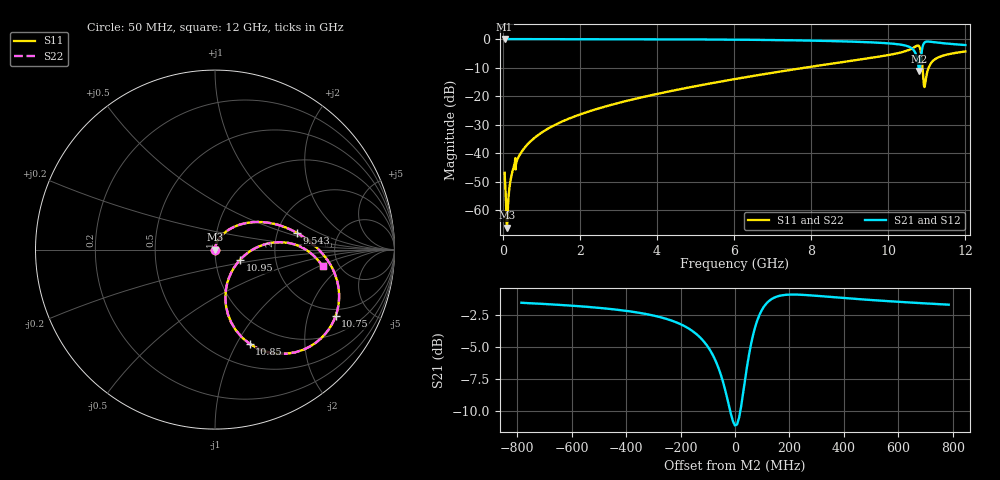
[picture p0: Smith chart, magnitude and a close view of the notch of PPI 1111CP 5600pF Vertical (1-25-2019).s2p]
# GHz S MA R 50
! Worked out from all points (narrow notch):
!   1601 points, 50 MHz to 12 GHz, reference 50 ohm
!   highest |S21| = 0.00 dB at 50 MHz (marker M1); lowest = -11.2 dB at 10.8 GHz (marker M2)
!   notch at M2: 11.0 dB deep, 131 MHz wide at half that depth
!   lowest |S11| = -66.1 dB at 109.8 MHz (marker M3), VSWR 1.00, Z = 50 - j0.0075 ohm
!   |S11| at or under -10 dB: start of sweep to 7.847 GHz; 10.89 GHz to 11.05 GHz (159.7 MHz wide, 1.46 % of centre)
!   |S22| runs from -66.1 to -2.2 dB; largest |S21 - S12| = 0
!   S11 on the Smith chart (normalised r, x): 50 MHz: 1.00, -0.01; 9.543 GHz: 2.59, +0.61; 10.75 GHz: 1.67, -3.02; 10.85 GHz: 0.74, -1.13; 10.95 GHz: 1.31, -0.16; 12 GHz: 3.74, -1.11
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0.05  0.00455 -85.4  0.9996 -0.0  0.9996 -0.0  0.00455 -85.4
0.10975  0.0004975 -8.7  0.9995 -0.6  0.9995 -0.6  0.0004975 -8.7
0.1545625  0.001804 70.8  0.9994 -1.0  0.9994 -1.0  0.001804 70.8
0.2068437  0.003451 78.0  0.9993 -1.4  0.9993 -1.4  0.003451 78.0
0.2665938  0.005178 80.2  0.9993 -1.8  0.9993 -1.8  0.005178 80.2
0.6026875  0.01331 81.5  0.9989 -4.2  0.9989 -4.2  0.01331 81.5
1.162844  0.02669 79.0  0.9982 -8.1  0.9982 -8.1  0.02669 79.0
2.044156  0.04886 73.6  0.9969 -14.3  0.9969 -14.3  0.04886 73.6
4.038312  0.1107 59.9  0.991 -28.8  0.991 -28.8  0.1107 59.9
6.025  0.1996 44.6  0.976 -44.4  0.976 -44.4  0.1996 44.6
8.019156  0.3293 27.1  0.9391 -62.0  0.9391 -62.0  0.3293 27.1
9.542781  0.4675 11.3  0.8769 -77.9  0.8769 -77.9  0.4675 11.3
10.01331  0.5264 5.2  0.8411 -83.9  0.8411 -83.9  0.5264 5.2
10.53613  0.6458 -7.2  0.7349 -94.6  0.7349 -94.6  0.6458 -7.2
10.74525  0.7675 -28.9  0.4626 -102.9  0.4626 -102.9  0.7675 -28.9
10.805  0.7431 -48.7  0.2764 -74.4  0.2764 -74.4  0.7431 -48.7
10.84981  0.5597 -69.8  0.476 -39.3  0.476 -39.3  0.5597 -69.8
10.89462  0.2735 -77.8  0.7524 -48.2  0.7524 -48.2  0.2735 -77.8
10.94691  0.1501 -22.7  0.8782 -61.7  0.8782 -61.7  0.1501 -22.7
11.03653  0.3026 6.6  0.9047 -74.0  0.9047 -74.0  0.3026 6.6
11.22325  0.4484 3.5  0.8743 -84.1  0.8743 -84.1  0.4484 3.5
12  0.6071 -8.9  0.7856 -98.1  0.7856 -98.1  0.6071 -8.9
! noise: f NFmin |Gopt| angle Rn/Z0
0.05  0.0004128  0.8784  0.2842  0.0007345
1.372  0.004377  0.7141  7.617  0.003008
2.701  0.00728  0.6733  14.81  0.004225
4.031  0.009959  0.6542  21.79  0.005297
5.36  0.01262  0.6475  28.5  0.006399
6.682  0.0154  0.6504  34.89  0.007651
8.012  0.01856  0.6624  41.04  0.009281
9.341  0.02304  0.6909  47.04  0.01228
10.67  0.1001  0.9113  54.75  0.1961
12  0.03108  0.7261  58.38  0.01732
